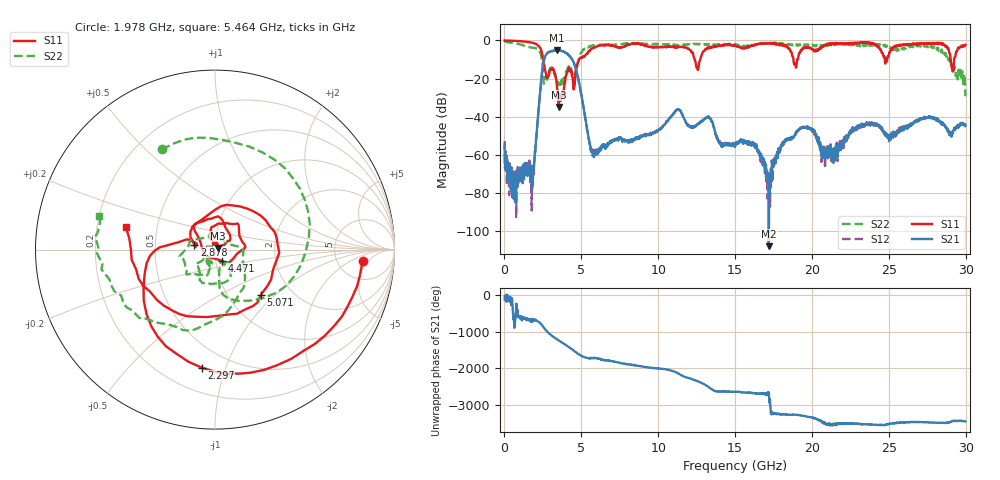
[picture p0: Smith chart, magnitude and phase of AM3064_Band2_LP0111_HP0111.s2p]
# Hz S DB R 50.0
!freq dBS11 angS11 dBS21 angS21 dBS12 angS12 dBS22 angS22
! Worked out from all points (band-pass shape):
!   1600 points, 10 MHz to 29.98 GHz, reference 50 ohm
!   highest |S21| = -5.07 dB at 3.403 GHz (marker M1); lowest = -107.9 dB at 17.2 GHz (marker M2)
!   |S21| within 3 dB of the highest: 2.666 GHz to 4.214 GHz (1.548 GHz wide, 45 % of centre)
!   lowest |S11| = -34.9 dB at 3.534 GHz (marker M3), VSWR 1.04, Z = 51.6 + j0.968 ohm
!   |S11| at or under -10 dB: 2.534 GHz to 4.864 GHz (2.331 GHz wide, 63 % of centre); 12.37 GHz to 12.73 GHz (357.9 MHz wide, 2.85 % of centre); 18.8 GHz to 19.05 GHz (250.7 MHz wide, 1.32 % of centre)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
!   |S22| runs from -29.3 to -0.2 dB; largest |S21 - S12| = 0.019
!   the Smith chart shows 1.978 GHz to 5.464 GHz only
!   S11 on the Smith chart (normalised r, x): 1.978 GHz: 8.98, -3.54; 2.297 GHz: 0.35, -0.83; 2.878 GHz: 0.79, +0.05; 4.471 GHz: 1.07, -0.13; 5.071 GHz: 1.42, -0.81; 5.464 GHz: 0.33, +0.11
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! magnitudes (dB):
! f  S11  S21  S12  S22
! 10 MHz  0.0  -55.4  -52.8  -0.2
! 628.5 MHz  -0.2  -75.5  -70.9  -1.5
! 1.978 GHz  -1.7  -58.1  -61.0  -4.0
! 2.297 GHz  -3.6  -29.1  -29.1  -5.9
! 2.878 GHz  -18.5  -6.1  -6.1  -17.5
! 3.403 GHz  -23.2  -5.1  -5.3  -21.8
! 3.534 GHz  -34.9  -5.3  -5.2  -22.6
! 4.471 GHz  -22.9  -11.1  -10.9  -20.4
! 5.015 GHz  -9.3  -29.2  -29.2  -6.4
! 5.071 GHz  -8.9  -31.9  -31.8  -5.6
! 5.464 GHz  -5.8  -50.7  -50.9  -3.5
! 10 GHz  -3.6  -47.1  -47.3  -2.0
! 11.31 GHz  -3.2  -36.2  -36.1  -2.6
! 15 GHz  -2.7  -54.7  -55.9  -2.1
! 16.3 GHz  -2.1  -56.4  -55.0  -2.3
! 17.2 GHz  -1.6  -107.9  -76.2  -1.7
! 18.29 GHz  -2.9  -53.0  -53.3  -2.3
! 19.99 GHz  -4.2  -46.7  -46.6  -2.3
! 21.34 GHz  -2.0  -63.2  -59.8  -2.1
! 25 GHz  -7.9  -49.8  -50.9  -3.1
! 28.31 GHz  -1.8  -42.6  -42.3  -4.6
! 29.98 GHz  -2.3  -44.4  -44.3  -29.3
